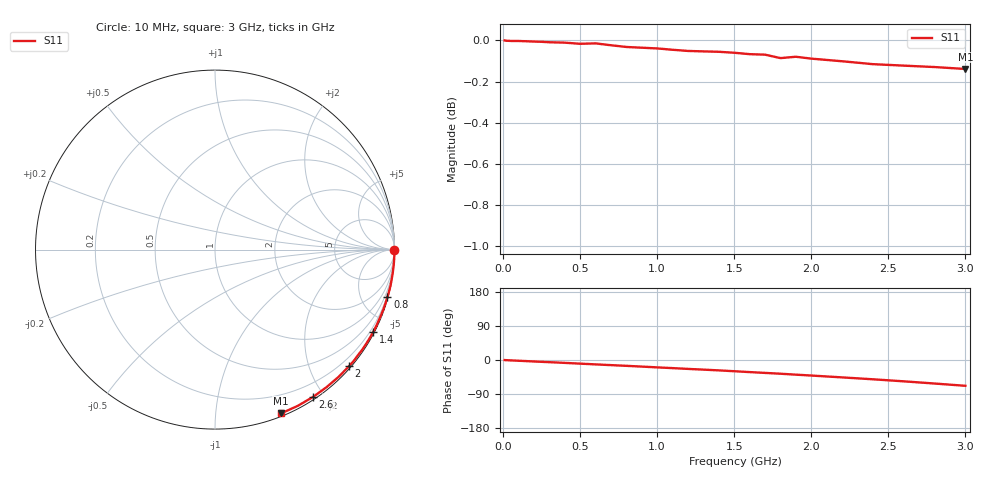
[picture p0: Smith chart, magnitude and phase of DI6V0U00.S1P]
! SIEMENS Small Signal Semiconductors
! BAV99
! Silicon Switching Diode in SOT23
! VR = 6 V
! S-Parameters:  May  1995
# GHz  S  MA  R  50
!  f  S11
! GHz  MAG  ANG
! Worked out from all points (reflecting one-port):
!   30 points, 10 MHz to 3 GHz, reference 50 ohm
!   lowest |S11| = -0.1 dB at 3 GHz (marker M1), VSWR 125.18, Z = 1.27 - j74 ohm
!   phase of S11 starts at -0 deg and turns -68 deg over the sweep
!   S11 on the Smith chart (normalised r, x): 10 MHz: open; 800 MHz: 0.10, -7.39; 1.4 GHz: 0.06, -4.10; 2 GHz: 0.04, -2.67; 2.6 GHz: 0.03, -1.87; 3 GHz: 0.03, -1.48
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0.01  1 -0.2
0.1  0.9997 -2.0
0.15  0.9995 -2.9
0.2  0.9994 -3.9
0.25  0.9992 -4.8
0.3  0.999 -5.7
0.4  0.9988 -7.6
0.5  0.9981 -9.6
0.6  0.9984 -11.6
0.7  0.9973 -13.5
0.8  0.9963 -15.4
0.9  0.9959 -17.4
1  0.9955 -19.5
1.1  0.9948 -21.4
1.2  0.9941 -23.5
1.3  0.9939 -25.4
1.4  0.9937 -27.4
1.5  0.9931 -29.6
1.6  0.9923 -31.9
1.7  0.9921 -34.1
1.8  0.9902 -36.2
1.9  0.9909 -38.7
2  0.9899 -41.0
2.2  0.9884 -45.9
2.4  0.9868 -50.9
2.6  0.986 -56.3
2.8  0.9852 -62.1
3  0.9841 -68.1
